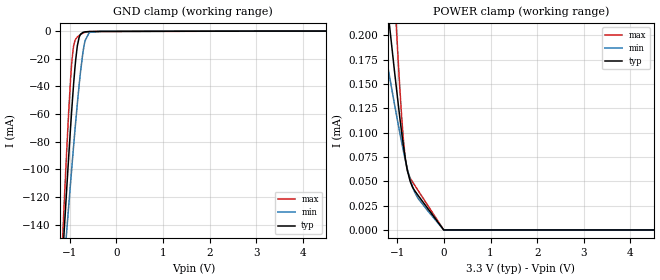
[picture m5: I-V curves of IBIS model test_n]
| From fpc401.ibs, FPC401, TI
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|   test_n Model
[Model]   test_n
Model_type   Input
Vinl = 0.8
Vinh = 2.0
|   typ   min   max
|   (nom PVT)   (fast PVT)   (slow PVT)
C_comp   1.056e-12   1.054e-12   1.064e-12
| Where nom  PVT is Nominal Process, 3.3V, 27C
|   Fast PVT is Strong Process,  3.6V, -40C
|   Slow PVT is Weak Process,   3V, 125C
[Voltage Range]   3.3   3   3.6
|Junction Temperature
[Temperature Range]   27   125   -40
[Power Clamp Reference]   3.3   3   3.6
[GND Clamp Reference]   0   0   0
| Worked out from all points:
|   GND clamp passes 1 mA (typ) near -0.72 V on its own axis
[GND Clamp]
|   Voltage   I(typ)   I(min)   I(max)
-3.3V     -1.497A    -1.178A    -1.889A
-1.197V   -189.4mA   -202mA     -182.1mA
-1.115V   -141.8mA   -166mA     -121mA
-1.076V   -119.7mA   -149.1mA   -93.29mA
-985.2mV  -70.83mA   -110.7mA   -36.16mA
-924mV    -41.13mA   -85.64mA   -12.21mA
-838.2mV  -10.77mA   -52.65mA   -4.3mA
-720mV    -986.9uA   -15.96mA   -1.546mA
-672mV    -556.6uA   -6.981mA   -923.9uA
-582mV    -301.4uA   -942.3uA   -410.8uA
-330mV    -233.9uA   -192uA     -289.6uA
6.6V      0A         0A         0A
[POWER Clamp]
|   Voltage   I(typ)   I(min)   I(max)
-3.3V     1.207mA    765.2uA    2.408mA
-1.37V    301.9uA    213.7uA    529.6uA
-1.188V   219.4uA    163.6uA    358.5uA
-1.056V   161.5uA    128.2uA    238.7uA
-960mV    121.3uA    103.4uA    157.2uA
-864.6mV  85.16uA    80.14uA    90.59uA
-826.8mV  72.99uA    71.6uA     73.26uA
-786mV    62.04uA    63.05uA    61.53uA
-715.2mV  48.87uA    50.4uA     52.66uA
-558mV    35.78uA    32.63uA    40.88uA
-3.3mV    0A         17.47nA    44.25nA
6.6V      0A         0A         0A
